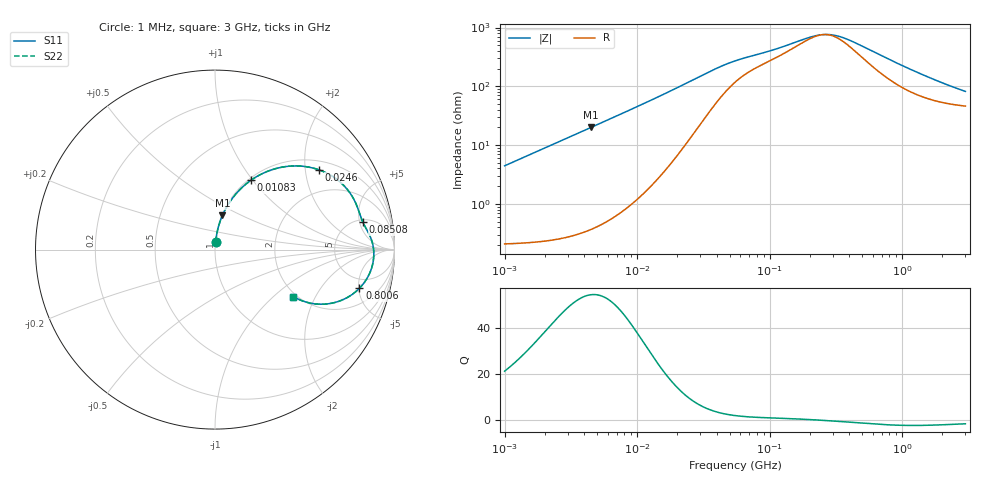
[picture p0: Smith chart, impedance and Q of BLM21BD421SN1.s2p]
! BLM21BD421SN1
# Hz S RI R 50
!Freq.(Hz) S11(Real) S11(Imag) S21(Real) S21(Imag) S12(Real) S12(Imag) S22(Real) S22(Imag)
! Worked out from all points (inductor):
!   401 points, 1 MHz to 3 GHz, reference 50 ohm
!   read as one part in series: L = 705 nH near 1.041 MHz
!   highest Q = 54.5 at 4.487 MHz (marker M1), where L = 707 nH
!   self-resonance near 254.3 MHz
!   S11 on the Smith chart (normalised r, x): 1 MHz: 1.00, +0.09; 10.83 MHz: 1.03, +0.98; 24.6 MHz: 1.24, +2.36; 85.08 MHz: 5.50, +5.61; 800.6 MHz: 3.61, -5.08; 3 GHz: 1.92, -1.36
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1000000  0.00402 0.044  0.996 -0.044  0.996 -0.044  0.00402 0.044
2055611  0.0105 0.0899  0.9895 -0.0899  0.9895 -0.0899  0.0105 0.0899
3823119  0.0309 0.164  0.9691 -0.164  0.9691 -0.164  0.0309 0.164
4487043  0.0415 0.1905  0.9585 -0.1905  0.9585 -0.1905  0.0415 0.1905
7254166  0.1 0.2899  0.9 -0.2899  0.9 -0.2899  0.1 0.2899
1.082539e7  0.2 0.386  0.8 -0.386  0.8 -0.386  0.2 0.386
1.461624e7  0.3176 0.4451  0.6824 -0.4451  0.6824 -0.4451  0.3176 0.4451
1.896016e7  0.445 0.4663  0.555 -0.4663  0.555 -0.4663  0.445 0.4663
2.459509e7  0.5774 0.4451  0.4226 -0.4451  0.4226 -0.4451  0.5774 0.4451
3.597591e7  0.7262 0.348  0.2738 -0.348  0.2738 -0.348  0.7262 0.348
5.477226e7  0.7962 0.2287  0.2038 -0.2287  0.2038 -0.2287  0.7962 0.2287
8.507507e7  0.8238 0.1521  0.1762 -0.1521  0.1762 -0.1521  0.8238 0.1521
2.094008e8  0.8785 0.0309  0.1215 -0.0309  0.1215 -0.0309  0.8785 0.0309
2.662515e8  0.8842 -0.00756  0.1158 0.00756  0.1158 0.00756  0.8842 -0.00756
3.318279e8  0.8839 -0.0452  0.1161 0.0452  0.1161 0.0452  0.8839 -0.0452
3.973271e8  0.8791 -0.0779  0.1209 0.0779  0.1209 0.0779  0.8791 -0.0779
5.258324e8  0.8616 -0.132  0.1384 0.132  0.1384 0.132  0.8616 -0.132
8.005644e8  0.8043 -0.216  0.1957 0.216  0.1957 0.216  0.8043 -0.216
1.147801e9  0.7194 -0.276  0.2806 0.276  0.2806 0.276  0.7194 -0.276
1.54974e9  0.6284 -0.3022  0.3716 0.3022  0.3716 0.3022  0.6284 -0.3022
2.092429e9  0.5336 -0.2987  0.4664 0.2987  0.4664 0.2987  0.5336 -0.2987
3e9  0.4366 -0.2616  0.5634 0.2616  0.5634 0.2616  0.4366 -0.2616
